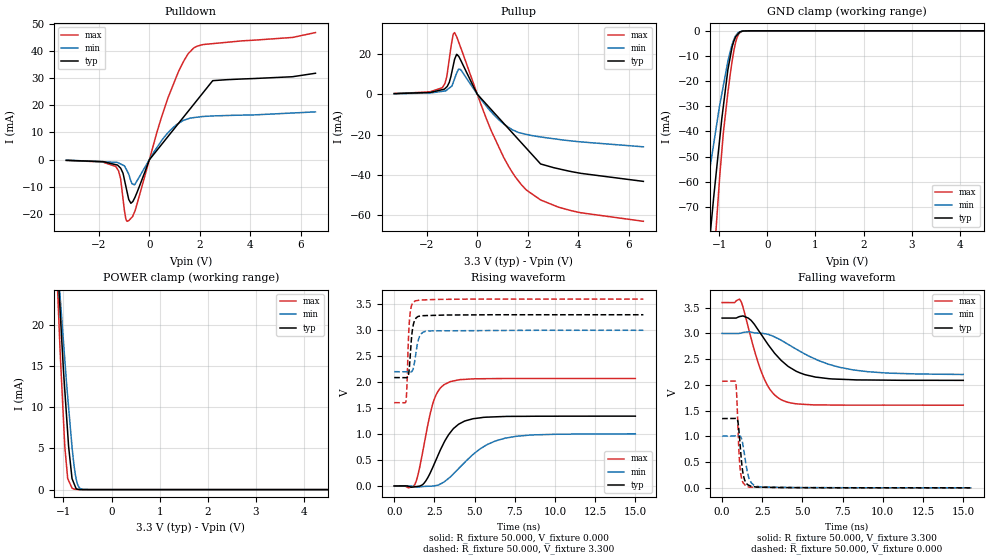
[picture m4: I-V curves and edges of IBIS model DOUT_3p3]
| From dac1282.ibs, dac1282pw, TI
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[Model] DOUT_3p3
Model_type   3-state
Polarity   Inverting
Vmeas = 1.65
Vref = 1.65
Cref = 2pF
Rref = 50
|   typ   min   max
|   (nom PVT)   (Fast PVT)   (slow PVT)
|   BUFFER OUTPUT TURNED HIGH
C_comp   2.249E-12   1.730E-12   2.806E-12
|   BUFFER OUTPUT LOW
|C_comp   2.399E-12   1.845E-12   2.993E-12
|   BUFFER HIGH Z STATE
|C_comp   2.260E-12   1.703E-12   2.821E-12
| Where   nom PVT is  Nominal Process, 3.3V, 30C
|   Fast PVT is Strong Process, 3.6V, -40C
|   Slow PVT is Weak Process, 3.0V, 88C
|C_comp - from L-C Tank method, L = 1nH, peak frequency
[Voltage Range]   3.3   3   3.6
[Temperature Range]   30   88   -40
[Pullup Reference]   3.3   3   3.6
[Pulldown Reference]   0   0   0
[Power Clamp Reference]   3.3   3   3.6
[GND Clamp Reference]   0   0   0
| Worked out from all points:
|   slope of the pulldown table from 0 to 0.495 V, typ, clamps not added: 86.2 ohm
|   slope of the pullup table from 0 to 0.495 V, typ, clamps not added: 72.5 ohm
|   GND clamp passes 1 mA (typ) near -0.60 V on its own axis
|   POWER clamp passes 1 mA (typ) near -0.80 V on its own axis
|   falling waveform, R_fixture 50.000, V_fixture 3.300: 20-80 % time 1.99ns typ, 3.25ns min, 1.24ns max; typ from 3.3 V to 2.09 V
|   rising waveform, R_fixture 50.000, V_fixture 0.000: 20-80 % time 1.34ns typ, 2.25ns min, 856ps max; typ from 0.001 V to 1.35 V
|   rising waveform, R_fixture 50.000, V_fixture 3.300: 20-80 % time 206ps typ, 279ps min, 151ps max; typ from 2.09 V to 3.3 V
|   falling waveform, R_fixture 50.000, V_fixture 0.000: 20-80 % time 251ps typ, 348ps min, 181ps max; typ from 1.35 V to 0.001 V
[Pulldown]
|   Voltage   I(typ)   I(min)   I(max)
-3.3V     -288.2uA   -204.7uA   -310.5uA
-1.339V   -1.878mA   -1.017mA   -2.538mA
-1.15V    -3.111mA   -1.593mA   -6.815mA
-1.047V   -5.08mA    -2.061mA   -14.53mA
-936.9mV  -9.794mA   -3.272mA   -21.84mA
-820.6mV  -14.73mA   -5.399mA   -22.55mA
-587.1mV  -14.18mA   -9.268mA   -19.26mA
-2.819mV  -72.38uA   -46.5uA    -98.27uA
739mV     8.538mA    9.904mA    22.84mA
1.756V    20.34mA    15.48mA    41.16mA
2.512V    29.11mA    16.1mA     42.78mA
6.59V     31.85mA    17.6mA     46.86mA
[GND Clamp]
|   Voltage   I(typ)   I(min)   I(max)
-3.3V     -564.8mA   -401.8mA   -784mA
-1.469V   -140.1mA   -92.84mA   -201.5mA
-1.325V   -108.7mA   -72.54mA   -156mA
-1.218V   -86.93mA   -57.62mA   -123.2mA
-1.105V   -64.17mA   -43.62mA   -89.56mA
-1V       -44.7mA    -30.52mA   -60.41mA
-914.6mV  -29.88mA   -21.73mA   -40.49mA
-821.3mV  -15.5mA    -12.14mA   -24.59mA
-694.9mV  -4.027mA   -3.394mA   -7.747mA
-608.3mV  -1.215mA   -697.8uA   -1.738mA
-1.859mV  0A         0A         0A
6.59V     0A         0A         0A
[Pullup]
|   Voltage   I(typ)   I(min)   I(max)
-3.3V     365uA      283.2uA    421.3uA
-1.388V   2.36mA     1.496mA    3.383mA
-1.214V   3.723mA    2.151mA    8.791mA
-1.113V   6.01mA     3.131mA    17.65mA
-905.3mV  17.33mA    7.692mA    30.74mA
-667.3mV  17.17mA    12.36mA    23.47mA
-2.819mV  70.81uA    50.24uA    100.2uA
553.2mV   -7.6mA     -8.764mA   -18.12mA
1.247V    -17.18mA   -16.45mA   -35.93mA
1.905V    -26.25mA   -19.78mA   -47.03mA
2.512V    -34.62mA   -21.2mA    -52.49mA
6.59V     -43.28mA   -26.09mA   -63.14mA
[POWER Clamp]
|   Voltage   I(typ)   I(min)   I(max)
-3.3V     287.4mA    234.7mA    365.7mA
-1.139V   28.93mA    29.29mA    26.64mA
-1.087V   23.5mA     24.82mA    19.26mA
-1.068V   21.63mA    23.38mA    16.71mA
-968.5mV  11.78mA    15.52mA    4.998mA
-911.5mV  6.852mA    11.26mA    1.345mA
-893.2mV  5.273mA    10.03mA    1.109mA
-821.3mV  1.336mA    5.157mA    177.8uA
-787.1mV  841.6uA    3.307mA    76.79uA
-708.5mV  44.69uA    679.2uA    19.36uA
-601mV    5.712uA    28.5uA     480.5nA
6.59V     0A         0A         0A
[Ramp]
R_load = 50
|   typ   min   max
dV/dt_r   0.918905/1.33277e-009  0.603262/2.24021e-009   1.24254/8.55015e-010
dV/dt_f   0.846857/1.96978e-009  0.478407/3.22935e-009   1.19615/1.23724e-009
[Falling Waveform]
R_fixture = 50.000
V_fixture = 3.300
V_fixture_min = 3.000
V_fixture_max = 3.600
C_fixture = 0.000
|  time   V(typ)   V(min)   V(max)
0s        3.299V     3V         3.6V
1.128ns   3.33V      3.004V     3.649V
1.295ns   3.341V     3.018V     3.517V
1.798ns   3.256V     3.027V     2.911V
2.522ns   2.94V      3V         2.189V
3.132ns   2.671V     2.952V     1.85V
3.738ns   2.459V     2.856V     1.703V
5.185ns   2.197V     2.595V     1.621V
8.106ns   2.101V     2.294V     1.607V
15ns      2.089V     2.203V     1.606V
[Rising Waveform]
R_fixture = 50.000
V_fixture = 0.000
V_fixture_min = 0.000
V_fixture_max = 0.000
C_fixture = 0.000
|  time   V(typ)   V(min)   V(max)
0s        1.255mV    66.77nV    92.6nV
1.282ns   -14.74mV   -10.9mV    29.1mV
1.488ns   -6.01mV    -20.41mV   227.4mV
1.865ns   57.38mV    -7.317mV   810.1mV
2.465ns   406.1mV    379uV      1.648V
2.939ns   737mV      50.41mV    1.91V
3.504ns   1.036V     178.2mV    2.012V
4.533ns   1.265V     501.4mV    2.057V
6.849ns   1.339V     917.9mV    2.071V
15ns      1.346V     1.005V     2.071V
[Rising Waveform]
R_fixture = 50.000
V_fixture = 3.300
V_fixture_min = 3.000
V_fixture_max = 3.600
C_fixture = 0.000
|  time   V(typ)   V(min)   V(max)
0s        2.089V     2.203V     1.606V
724.4ps   2.087V     2.2V       1.622V
785.9ps   2.087V     2.2V       1.887V
877.9ps   2.123V     2.2V       2.765V
976.5ps   2.415V     2.199V     3.288V
1.118ns   2.971V     2.212V     3.508V
1.316ns   3.214V     2.485V     3.567V
1.575ns   3.273V     2.88V      3.581V
1.944ns   3.283V     2.98V      3.586V
15.5ns    3.299V     3V         3.6V
[Falling Waveform]
R_fixture = 50.000
V_fixture = 0.000
V_fixture_min = 0.000
V_fixture_max = 0.000
C_fixture = 0.000
|  time   V(typ)   V(min)   V(max)
0s        1.346V     1.005V     2.071V
838.4ps   1.35V      1.01V      2.056V
908.9ps   1.346V     1.01V      1.79V
987.6ps   1.277V     1.01V      1.164V
1.117ns   849.3mV    1.006V     383.2mV
1.277ns   325.3mV    865.5mV    120.2mV
1.483ns   101.4mV    459.2mV    35.35mV
1.82ns    30.9mV     95.72mV    13.28mV
2.451ns   13.18mV    17.45mV    10.96mV
15.5ns    1.255mV    22.85nV    1.682nV
